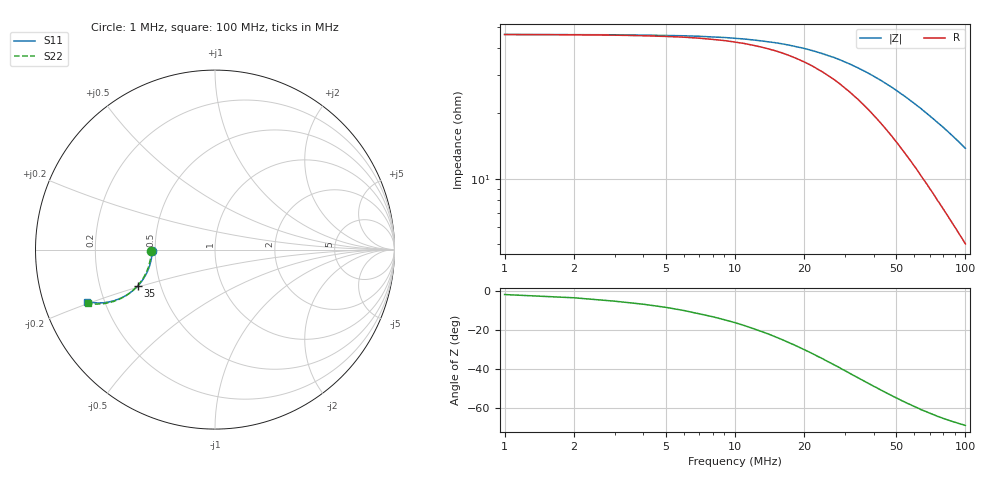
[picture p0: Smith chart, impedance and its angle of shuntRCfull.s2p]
# Hz S RI R 50.0
! written by SimSmith version 18.3b
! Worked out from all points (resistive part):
!   100 points, 1 MHz to 100 MHz, reference 50 ohm
!   read as one part in shunt: R = 46.1 ohm at 1 MHz
!   S11 on the Smith chart (normalised r, x): 1 MHz: 0.48, -0.01; 35 MHz: 0.37, -0.19; 100 MHz: 0.14, -0.19
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1000000  -0.3514 -0.00742  0.6508 -0.0067  0.6502 -0.00689  -0.3563 -0.0055
2000000  -0.3501 -0.0135  0.6495 -0.0131  0.6498 -0.0136  -0.3562 -0.013
3000000  -0.3509 -0.0199  0.6495 -0.0206  0.6495 -0.0203  -0.3561 -0.0193
6000000  -0.3531 -0.0395  0.648 -0.0398  0.648 -0.0395  -0.3579 -0.0384
9000000  -0.3558 -0.0588  0.645 -0.0592  0.645 -0.0592  -0.361 -0.0578
1.3e7  -0.3623 -0.0836  0.6385 -0.0847  0.6383 -0.085  -0.3668 -0.0828
1.8e7  -0.3729 -0.1136  0.6278 -0.1153  0.6277 -0.1154  -0.377 -0.1129
2.7e7  -0.399 -0.1633  0.6025 -0.1657  0.6023 -0.166  -0.4023 -0.1636
3.4e7  -0.4251 -0.1968  0.5771 -0.2002  0.577 -0.2003  -0.4275 -0.1974
3.5e7  -0.429 -0.2014  0.5726 -0.2046  0.5727 -0.2049  -0.4314 -0.2019
4e7  -0.4499 -0.2218  0.5525 -0.2259  0.5522 -0.2262  -0.4518 -0.2226
4.3e7  -0.463 -0.2324  0.5395 -0.237  0.5393 -0.237  -0.4645 -0.2338
5.1e7  -0.4994 -0.2573  0.5037 -0.2626  0.5036 -0.2628  -0.5002 -0.2591
5.6e7  -0.5229 -0.2694  0.481 -0.2759  0.4808 -0.2763  -0.5233 -0.272
6.3e7  -0.5555 -0.2822  0.4483 -0.2896  0.448 -0.2899  -0.5552 -0.285
6.4e7  -0.564 -0.2857  0.4455 -0.2933  0.4438 -0.2921  -0.5599 -0.2871
6.5e7  -0.5644 -0.2853  0.4388 -0.293  0.4385 -0.2933  -0.5641 -0.2886
6.7e7  -0.5744 -0.2877  0.4301 -0.2959  0.4299 -0.2964  -0.5736 -0.2911
7.7e7  -0.6193 -0.296  0.3861 -0.3059  0.3857 -0.3063  -0.6173 -0.3003
8.4e7  -0.6487 -0.2971  0.357 -0.3091  0.3565 -0.3095  -0.6457 -0.3028
9.4e7  -0.6888 -0.2939  0.3176 -0.3084  0.3172 -0.3084  -0.6848 -0.3021
1e8  -0.711 -0.29  0.2957 -0.3062  0.2953 -0.3064  -0.7066 -0.2988
